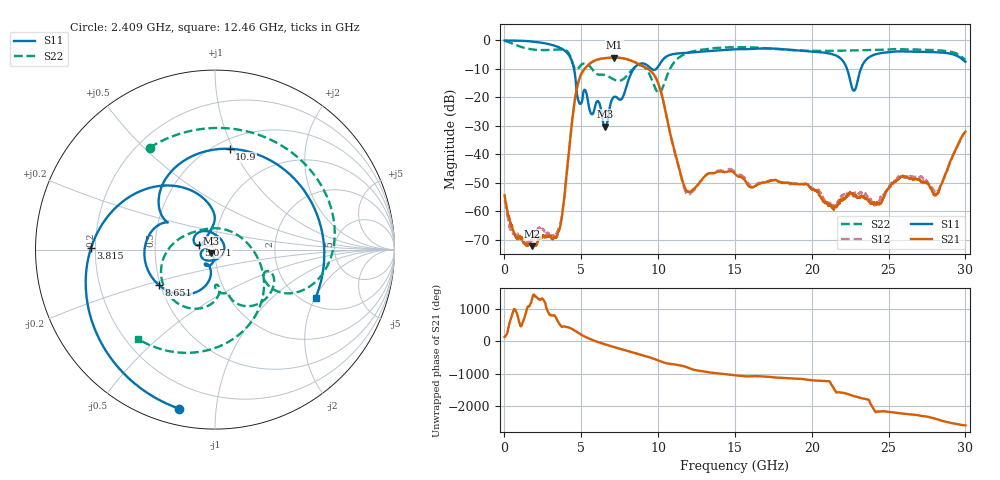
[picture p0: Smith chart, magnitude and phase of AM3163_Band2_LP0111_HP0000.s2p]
!Agilent Technologies,E8364B,MY43040894,A.07.50.67
!Agilent E8364B: A.07.50.67
!Date: Thursday, August 20, 2020 12:05:58
!Correction: S11(Full 2 Port(1,2))
!S21(Full 2 Port(1,2))
!S12(Full 2 Port(1,2))
!S22(Full 2 Port(1,2))
!S2P File: Measurements: S11, S21, S12, S22:
# Hz S  dB  R 50
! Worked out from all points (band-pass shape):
!   3201 points, 10 MHz to 30 GHz, reference 50 ohm
!   highest |S21| = -6.04 dB at 7.142 GHz (marker M1); lowest = -72.2 dB at 1.819 GHz (marker M2)
!   |S21| within 3 dB of the highest: 5.377 GHz to 9.023 GHz (3.646 GHz wide, 50.6 % of centre)
!   lowest |S11| = -30.2 dB at 6.561 GHz (marker M3), VSWR 1.06, Z = 47.7 - j1.88 ohm
!   |S11| at or under -10 dB: 4.527 GHz to 8.412 GHz (3.886 GHz wide, 60.1 % of centre); 9.571 GHz to 9.88 GHz (309.2 MHz wide, 3.18 % of centre); 22.3 GHz to 23.2 GHz (899.8 MHz wide, 3.96 % of centre)
!   |S22| runs from -18.5 to -0.2 dB; largest |S21 - S12| = 0.004
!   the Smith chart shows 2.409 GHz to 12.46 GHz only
!   S11 on the Smith chart (normalised r, x): 2.409 GHz: 0.08, -0.79; 3.815 GHz: 0.18, +0.01; 5.071 GHz: 0.84, +0.04; 8.651 GHz: 0.49, -0.22; 10.9 GHz: 0.58, +0.97; 12.46 GHz: 2.32, -2.02
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1e7  -0.04 -3.0  -54.38 126.5  -56.08 34.0  -0.22 -9.6
7.128906e8  -0.07 -29.4  -68.73 -131.3  -68.18 -131.1  -1.56 -91.2
1.818772e9  -0.42 -76.4  -72.22 -101.5  -69.73 5.2  -3.19 166.6
2.4092e9  -0.83 -102.9  -69.25 -140.1  -66.23 -105.7  -3.41 122.7
3.814981e9  -3.21 179.3  -58.64 86.3  -58.44 87.2  -3.26 19.6
5.014581e9  -21.91 155.8  -11.65 -168.7  -11.66 -169.0  -8.50 -28.9
5.070812e9  -20.72 164.6  -11.10 176.3  -11.11 176.0  -8.32 -32.1
5.923653e9  -22.60 -124.7  -6.98 -0.4  -7.00 -0.5  -11.48 -72.8
6.560941e9  -30.24 -140.2  -6.23 -102.1  -6.25 -102.2  -12.18 -80.9
7.141997e9  -19.81 -117.9  -6.04 175.5  -6.05 175.5  -13.78 -89.8
7.8074e9  -18.49 -101.5  -6.39 85.5  -6.42 85.6  -13.28 -83.7
8.650869e9  -8.64 -147.8  -8.07 -25.8  -8.07 -25.8  -8.94 -114.8
1.000979e10  -9.13 147.6  -15.12 123.6  -15.07 123.2  -18.43 98.5
1.090012e10  -4.92 81.7  -35.30 12.1  -35.49 10.3  -8.80 -42.1
1.245585e10  -4.14 -25.5  -51.45 -176.2  -51.74 -175.1  -3.64 -130.4
1.5005e10  -3.16 -142.4  -46.83 22.9  -46.21 24.0  -2.40 137.2
1.772284e10  -2.94 94.3  -49.18 -43.7  -49.40 -42.4  -3.07 32.7
2.000958e10  -3.92 -26.6  -52.32 -126.2  -51.75 -116.9  -3.68 -49.6
2.274617e10  -17.66 -109.6  -54.45 105.3  -54.38 113.0  -3.53 -127.6
2.500479e10  -4.17 -151.3  -52.01 -19.4  -51.80 -23.7  -3.23 176.6
2.809751e10  -4.17 110.7  -54.18 120.4  -53.09 127.4  -3.43 93.8
3e10  -7.49 38.4  -32.08 -78.0  -32.12 -78.5  -6.82 35.2
